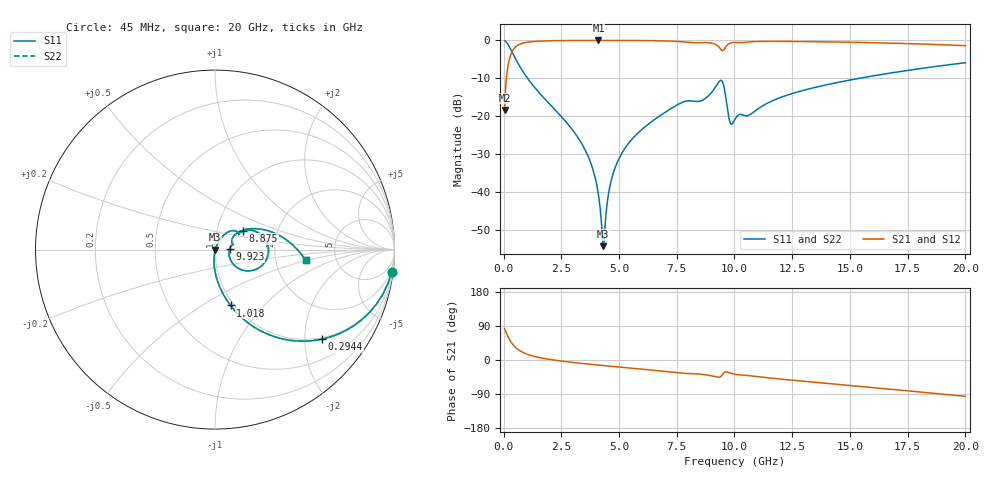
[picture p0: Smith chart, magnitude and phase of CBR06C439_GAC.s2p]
! S-parameter model data by Modelithics Inc.  support@modelithics.com 813-866-6335  Tampa FL USA
! S-Parameter data specifications:
! Substrate: 20-mil Rogers 4350B, substrate thickness, H=0.508mm, Dielectric constant, Er=3.75
! PCB Mounting Pad Footprint: Pad width, PadW=0.85mm , Pad length, PadL=0.64mm , Pad gap, PadG (edge-to-edge)=0.62mm , Reference planes=1.9mm apart
#  GHz  S  MA  R 50
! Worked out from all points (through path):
!   801 points, 45 MHz to 20 GHz, reference 50 ohm
!   highest |S21| = -0.02 dB at 4.111 GHz (marker M1); lowest = -18.3 dB at 45 MHz (marker M2)
!   group delay of S21, straight-line fit = 15.6 ps
!   lowest |S11| = -54.2 dB at 4.31 GHz (marker M3), VSWR 1.00, Z = 50.2 - j0.09 ohm
!   |S11| at or under -10 dB: 1.039 GHz to 15.39 GHz (14.35 GHz wide, 175 % of centre)
!   |S22| runs from -54.2 to -0.1 dB; largest |S21 - S12| = 0
!   S11 on the Smith chart (normalised r, x): 45 MHz: 1, -16; 294.4 MHz: 0.96, -2.43; 1.018 GHz: 0.96, -0.67; 8.875 GHz: 1.33, +0.29; 9.923 GHz: 1.18, +0.01; 20 GHz: 2.98, -0.48
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0.045  0.9925 -7.2  0.1218 82.8  0.1218 82.8  0.9925 -7.2
0.294438  0.7781 -39.9  0.6276 50.1  0.6276 50.1  0.7781 -39.9
0.593762  0.5183 -60.7  0.8544 29.2  0.8544 29.2  0.5183 -60.7
1.017806  0.323 -74.5  0.9454 15.4  0.9454 15.4  0.323 -74.5
3.387462  0.04364 -96.9  0.9972 -9.0  0.9972 -9.0  0.04364 -96.9
3.83645  0.02153 -97.1  0.9978 -11.8  0.9978 -11.8  0.02153 -97.1
4.110831  0.009243 -92.0  0.9979 -13.5  0.9979 -13.5  0.009243 -92.0
4.310381  0.00196 -27.2  0.9979 -14.6  0.9979 -14.6  0.00196 -27.2
4.385212  0.003359 39.6  0.9978 -15.1  0.9978 -15.1  0.003359 39.6
4.63465  0.01324 64.6  0.9976 -16.5  0.9976 -16.5  0.01324 64.6
4.983862  0.02725 66.8  0.9971 -18.5  0.9971 -18.5  0.02725 66.8
5.6324  0.05293 64.8  0.9955 -22.2  0.9955 -22.2  0.05293 64.8
6.704981  0.09861 58.1  0.9886 -28.4  0.9886 -28.4  0.09861 58.1
8.875087  0.1869 33.6  0.9313 -40.3  0.9313 -40.3  0.1869 33.6
9.2243  0.2558 22.2  0.871 -44.7  0.871 -44.7  0.2558 22.2
9.448794  0.2951 -8.4  0.7381 -41.0  0.7381 -41.0  0.2951 -8.4
9.773062  0.09179 -27.8  0.9081 -33.4  0.9081 -33.4  0.09179 -27.8
9.922725  0.08117 2.5  0.935 -36.3  0.935 -36.3  0.08117 2.5
10.0225  0.09156 12.4  0.9384 -37.7  0.9384 -37.7  0.09156 12.4
13.36496  0.2356 29.7  0.9623 -58.1  0.9623 -58.1  0.2356 29.7
16.68248  0.3688 12.2  0.9211 -76.7  0.9211 -76.7  0.3688 12.2
20  0.5083 -6.7  0.8524 -95.9  0.8524 -95.9  0.5083 -6.7
